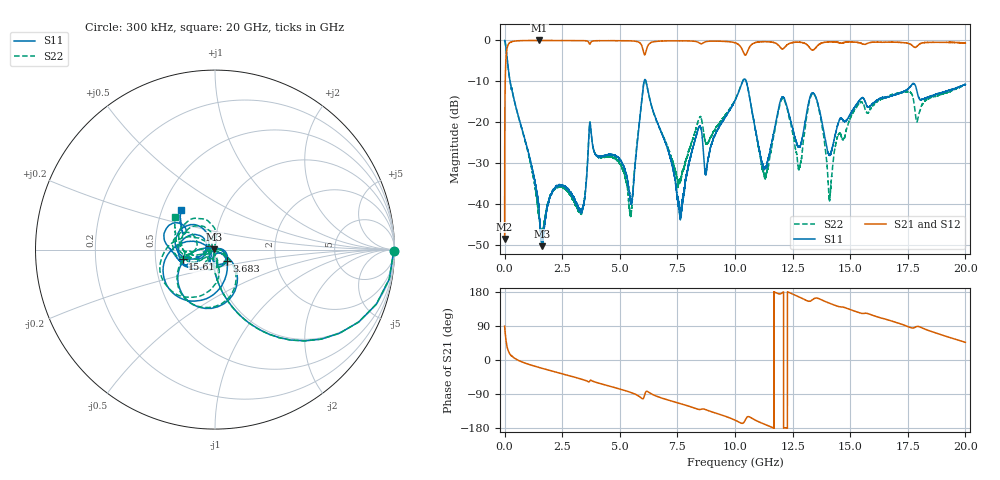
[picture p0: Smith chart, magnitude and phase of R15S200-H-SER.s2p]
!{R15S200}
!Johanson Technology Inc.
!www.johansontechnology.com
!Test Board Conditions:
!Substrate Type  RO4350B
!Substrate Thickness  20 mil
!Substrate Dk  3.66
!TL Type: GCPW
!TL Trace Width  34 mil
!TL Gap  10 mil
!Electrode orientation  Horizontal
!DUT TOPOLOGY	SERIES
!Mounting Pad LxW  26x52 mil
! Created Sat Feb  6 14:18:56 2021
# hz S ma R 50
! 2 Port Network Data from SP1.SP block
! freq  magS11  angS11  magS21  angS21  magS12  angS12  magS22  angS22
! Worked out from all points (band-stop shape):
!   20001 points, 300 kHz to 20 GHz, reference 50 ohm
!   highest |S21| = 0.00 dB at 1.512 GHz (marker M1); lowest = -48.6 dB at 300 kHz (marker M2)
!   |S21| within 3 dB of the highest: 80.34 MHz to 6.04 GHz (5.959 GHz wide, 195 % of centre); 10.52 GHz to end of sweep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
!   lowest |S11| = -50.3 dB at 1.623 GHz (marker M3), VSWR 1.01, Z = 49.7 + j0.0903 ohm
!   |S11| at or under -10 dB: 235 MHz to 6.056 GHz (5.821 GHz wide, 185 % of centre); 6.135 GHz to 10.34 GHz (4.2 GHz wide, 51 % of centre); 10.48 GHz to end of sweep
!   |S22| runs from -48.2 to 0.0 dB; largest |S21 - S12| = 0.015
!   S11 on the Smith chart (normalised r, x): 300 kHz: open; 3.683 GHz: 1.13, -0.15; 15.61 GHz: 0.69, -0.07; 20 GHz: 0.63, +0.30
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300000  0.9955 -0.5  0.003735 89.1  0.003688 90.0  0.9957 -0.4
1.633e8  0.4351 -66.1  0.8967 23.6  0.8975 23.5  0.4367 -66.1
1.5123e9  0.006534 -135.0  0.9995 -20.0  0.9986 -20.0  0.006503 -74.7
1.6233e9  0.003045 162.6  0.9984 -22.0  0.999 -22.0  0.003951 -20.7
3.3343e9  0.007903 43.0  0.9951 -50.4  0.9954 -50.4  0.007821 8.3
3.6833e9  0.09177 -43.9  0.9045 -56.9  0.9047 -56.9  0.09309 -53.5
5.4603e9  0.01133 -120.4  0.9886 -85.3  0.9877 -85.3  0.007311 -113.7
6.0623e9  0.3219 -88.8  0.6742 -96.1  0.6759 -96.1  0.3192 -91.6
6.6673e9  0.09343 -179.5  0.9792 -97.2  0.9783 -97.2  0.0933 -178.9
7.6333e9  0.007608 79.8  0.9889 -115.3  0.9895 -115.3  0.02035 -107.0
8.4053e9  0.08317 -44.8  0.9491 -130.1  0.9484 -130.1  0.1043 -88.7
8.7553e9  0.02492 -51.1  0.9683 -131.7  0.9684 -131.6  0.05434 -108.7
1.00003e10  0.184 -74.3  0.9366 -158.6  0.9357 -158.6  0.1881 -88.4
1.04843e10  0.3165 -155.8  0.6744 -153.7  0.6755 -153.8  0.3189 -164.1
1.13063e10  0.02838 -153.0  0.9667 -170.1  0.9675 -170.1  0.02049 -177.6
1.20673e10  0.2042 -173.8  0.7889 178.2  0.7881 178.1  0.1965 158.6
1.28123e10  0.04981 175.1  0.9497 165.6  0.9506 165.5  0.02858 154.4
1.33343e10  0.2257 169.1  0.7644 157.8  0.7646 157.6  0.2204 155.7
1.41143e10  0.03946 168.7  0.9619 149.5  0.9604 149.5  0.01152 149.7
1.56113e10  0.1874 -164.3  0.8951 122.9  0.894 123.2  0.1581 -176.8
1.66673e10  0.2051 -162.2  0.956 105.2  0.9459 105.1  0.2092 -168.8
2e10  0.2887 130.8  0.9309 46.6  0.9251 46.4  0.2891 140.7
